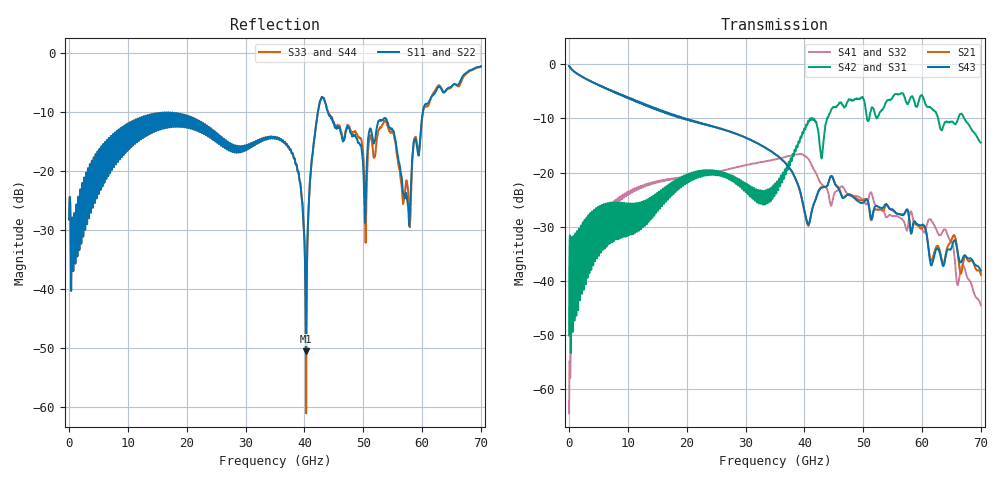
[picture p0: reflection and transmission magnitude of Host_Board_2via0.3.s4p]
! AWR Design Environment (8415) Fri Sep 21 17:00:08 2018
! Document = 'Host PCB'
! nPorts: 4, nXvals: 7001
# HZ S DB R 50
!Freq DBS11 AngS11 DBS12 AngS12 DBS13 AngS13 DBS14 AngS14
!	DBS21 AngS21 DBS22 AngS22 DBS23 AngS23 DBS24 AngS24
!	DBS31 AngS31 DBS32 AngS32 DBS33 AngS33 DBS34 AngS34
!	DBS41 AngS41 DBS42 AngS42 DBS43 AngS43 DBS44 AngS44
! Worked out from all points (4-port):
!   7000 points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, 10 MHz to 70 GHz, reference 50 ohm
!   strongest paths, dB at 10 MHz, 17.51 GHz, 35.01 GHz, 52.51 GHz, 70 GHz:
!     S43: -0.3, -9.4, -16.6, -26.3, -38.1
!     S21: -0.3, -9.4, -16.6, -26.9, -38.9
!     S42: -50.1, -22.4, -22.3, -9.6, -14.5
!     S31: -50.1, -22.4, -22.3, -9.6, -14.5
!     S41: -64.5, -21.2, -17.6, -26.3, -44.5
!     S32: -64.5, -21.2, -17.6, -26.3, -44.5
!   lowest |S11| = -50.5 dB at 40.29 GHz (marker M1), VSWR 1.01, Z = 49.7 - j0.0198 ohm
!   |S11| at or under -10 dB: start of sweep to 42.28 GHz; 44.02 GHz to 60.12 GHz (16.1 GHz wide, 30.9 % of centre)
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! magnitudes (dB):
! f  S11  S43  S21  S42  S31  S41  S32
! 10 MHz  -28.2  -0.3  -0.3  -50.1  -50.1  -64.5  -64.5
! 6.91 GHz  -17.1  -4.7  -4.7  -26.7  -26.7  -26.0  -26.0
! 36.04 GHz  -14.6  -17.5  -17.5  -20.5  -20.5  -17.3  -17.3
! 40.29 GHz  -50.5  -28.4  -28.6  -11.2  -11.2  -17.1  -17.1
! 42.93 GHz  -7.5  -22.8  -22.7  -17.4  -17.4  -22.2  -22.2
! 57.71 GHz  -27.4  -27.7  -27.8  -7.1  -7.1  -29.1  -29.1
! 70 GHz  -2.2  -38.1  -38.9  -14.5  -14.5  -44.5  -44.5
